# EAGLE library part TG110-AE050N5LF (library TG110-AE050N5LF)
Audio Transformers / Signal Transformers 10/100BASE-TX SMD AEC-Q200 16P 1-Port Source: Datasheet
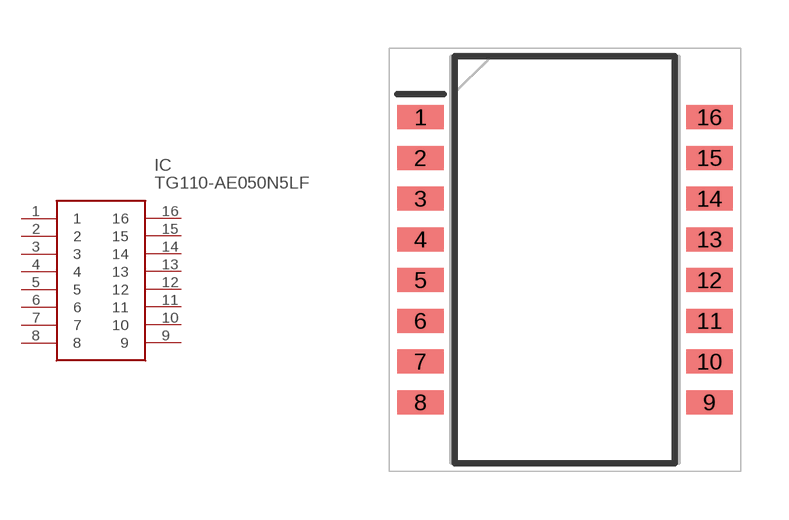
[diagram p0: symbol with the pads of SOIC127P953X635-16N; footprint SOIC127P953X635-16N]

Designator prefix IC

## TG110-AE050N5LF (Description: Audio Transformers / Signal Transformers 10/100BASE-TX SMD AEC-Q200 16P 1-Port; Height: 6.35mm; Manufacturer_Name: Halo Electronics; Manufacturer_Part_Number: TG110-AE050N5LF; Mouser_Part_Number: 493-TG110-AE050N5LF; Mouser_Price-Stock: https://www.mouser.co.uk/ProductDetail/HALO-Electronics/TG110-AE050N5LF?qs=8uu3sA0mUdvZuJUwPIBEMQ%3D%3D)  [SOIC127P953X635-16N]
1  1
2  2
3  3
4  4
5  5
6  6
7  7
8  8
9  9
10  10
11  11
12  12
13  13
14  14
15  15
16  16

## Footprint SOIC127P953X635-16N (pad centres in mm)
n2
smd 1.45 x 0.75: 1 -4.5,4.445; 2 -4.5,3.175; 3 -4.5,1.905; 4 -4.5,0.635; 5 -4.5,-0.635; 6 -4.5,-1.905; 7 -4.5,-3.175; 8 -4.5,-4.445; 9 4.5,-4.445; 10 4.5,-3.175; 11 4.5,-1.905; 12 4.5,-0.635; 13 4.5,0.635; 14 4.5,1.905; 15 4.5,3.175; 16 4.5,4.445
